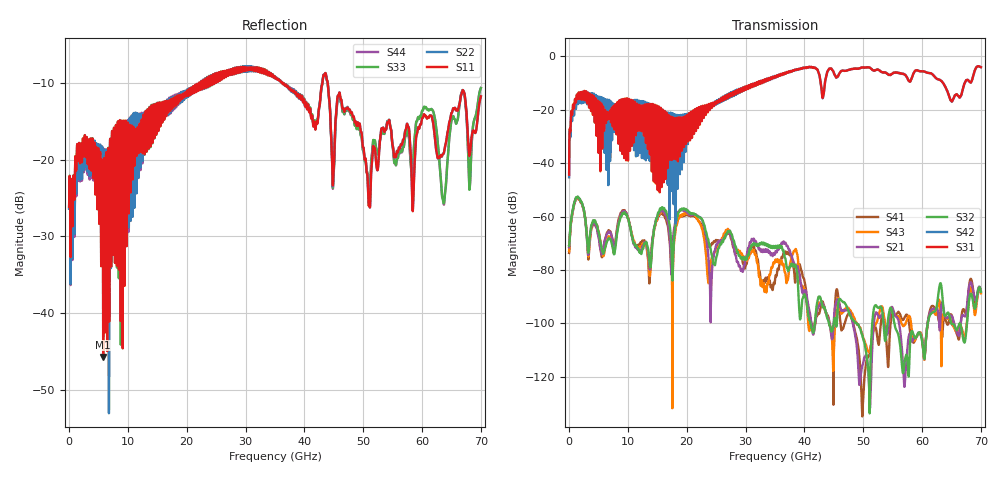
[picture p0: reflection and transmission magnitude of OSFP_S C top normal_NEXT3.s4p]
! AWR Design Environment (8415) Mon Jan 07 17:02:14 2019
! Document = 'OSFP Channel_S'
! nPorts: 4, nXvals: 7001
# HZ S DB R 50
!Freq DBS11 AngS11 DBS12 AngS12 DBS13 AngS13 DBS14 AngS14
!	DBS21 AngS21 DBS22 AngS22 DBS23 AngS23 DBS24 AngS24
!	DBS31 AngS31 DBS32 AngS32 DBS33 AngS33 DBS34 AngS34
!	DBS41 AngS41 DBS42 AngS42 DBS43 AngS43 DBS44 AngS44
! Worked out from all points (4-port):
!   7000 points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, 10 MHz to 70 GHz, reference 50 ohm
!   strongest paths, dB at 10 MHz, 17.51 GHz, 35.01 GHz, 52.51 GHz, 70 GHz:
!     S31: -44.3, -28.3, -7.4, -4.9, -4.0
!     S42: -45.3, -27.8, -7.4, -4.9, -4.0
!     S32: -70.9, -78.3, -71.5, -94.1, -88.2
!     S21: -71.5, -75.4, -73.9, -96.9, -87.8
!     S43: -73.0, -86.6, -76.7, -98.0, -88.7
!     S41: -73.6, -74.1, -83.7, -107.0, -88.4
!   lowest |S11| = -45.7 dB at 5.8 GHz (marker M1), VSWR 1.01, Z = 49.8 + j0.464 ohm
!   |S11| at or under -10 dB: start of sweep to 22.12 GHz; 36.24 GHz to 43.05 GHz (6.813 GHz wide, 17.2 % of centre); 43.96 GHz to end of sweep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
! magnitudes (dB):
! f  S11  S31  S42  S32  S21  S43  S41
! 10 MHz  -26.2  -44.3  -45.3  -70.9  -71.5  -73.0  -73.6
! 1.61 GHz  -19.1  -13.6  -15.0  -53.0  -53.2  -53.3  -53.5
! 5.8 GHz  -45.7  -18.8  -16.7  -73.7  -72.1  -74.6  -73.1
! 19.52 GHz  -11.7  -33.9  -37.4  -56.9  -57.4  -58.8  -59.3
! 24.09 GHz  -9.4  -17.6  -18.0  -72.8  -95.3  -77.3  -70.8
! 63.64 GHz  -19.2  -10.2  -10.1  -95.0  -94.2  -96.7  -98.7
! 70 GHz  -11.8  -4.0  -4.0  -88.2  -87.8  -88.7  -88.4
